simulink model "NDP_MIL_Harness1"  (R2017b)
settings: Solver=FixedStepDiscrete  StartTime=0.0  StopTime=70  FixedStep=0.01  RelTol=1e-3  EnableMultiTasking=on
undefined symbols (not defined in the file): sigbuilder_block

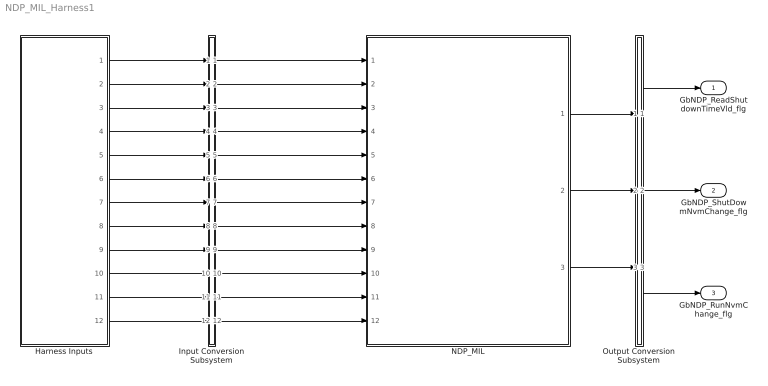
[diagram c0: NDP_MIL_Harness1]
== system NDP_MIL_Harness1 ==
  Harness Inputs : Subsystem  Tag=STV Subsys  LoadFcn=sigbuilder_block('load');  StartFcn=sigbuilder_block('start');  StopFcn=sigbuilder_block('stop');  ClipboardFcn=sigbuilder_block('clipboard');  mask(Sigbuilder block){tuvar=[0:10]}
      mask init:
      | if ~strcmp(get_param(bdroot(gcb),'SimulationStatus'),'stopped'),tuvar = sigbuilder_block('maskInit'); end
  Input Conversion Subsystem : Subsystem  Tag=__SLT_ICS__  Description=Signal spec. and routing
  NDP_MIL : ModelReference  ModelNameDialog=NDP_MIL  SimulationMode=Normal  ModelReferenceVersion='M115C124'
  Output Conversion Subsystem : Subsystem  Tag=__SLT_OCS__  Description=Signal spec. and routing
  GbNDP_ReadShutdownTimeVld_flg : Outport  OutDataTypeStr=boolean  PortDimensions=[1]
  GbNDP_ShutDowmNvmChange_flg : Outport  Port=2  OutDataTypeStr=boolean  PortDimensions=[1]
  GbNDP_RunNvmChange_flg : Outport  Port=3  OutDataTypeStr=boolean  PortDimensions=[1]
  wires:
  Harness Inputs/1(GbNVM_ReadTimeYrVld_flg) -> Input Conversion Subsystem/1(Inport_1)
  Harness Inputs/2(GbNVM_ReadTimeMonthVld_flg) -> Input Conversion Subsystem/2(Inport_2)
  Harness Inputs/3(GbNVM_ReadTimeDayVld_flg) -> Input Conversion Subsystem/3(Inport_3)
  Harness Inputs/4(GbNVM_ReadTimeHrVld_flg) -> Input Conversion Subsystem/4(Inport_4)
  Harness Inputs/5(GbNVM_ReadTimeMintVld_flg) -> Input Conversion Subsystem/5(Inport_5)
  Harness Inputs/6(GbNVM_ReadTimeSecVld_flg) -> Input Conversion Subsystem/6(Inport_6)
  Harness Inputs/7(GeMSM_BMUState_enum) -> Input Conversion Subsystem/7(Inport_7)
  Harness Inputs/8(GbACC_ACChrgFinish_flg) -> Input Conversion Subsystem/8(Inport_8)
  Harness Inputs/9(GbDCC_DCChrgFinish_flg) -> Input Conversion Subsystem/9(Inport_9)
  Harness Inputs/10(GeCTC_CtrCtlState_enum) -> Input Conversion Subsystem/10(Inport_10)
  Harness Inputs/11(GbDAS_HVSafetyNVMStore_flg) -> Input Conversion Subsystem/11(Inport_11)
  Harness Inputs/12(GbDAS_NormalNVMStore_flg) -> Input Conversion Subsystem/12(Inport_12)
  Output Conversion Subsystem/1(Outport_1) -> GbNDP_ReadShutdownTimeVld_flg/1
  Output Conversion Subsystem/2(Outport_2) -> GbNDP_ShutDowmNvmChange_flg/1
  Output Conversion Subsystem/3(Outport_3) -> GbNDP_RunNvmChange_flg/1
  Input Conversion Subsystem/1(Outport_1) -> NDP_MIL/1
  Input Conversion Subsystem/2(Outport_2) -> NDP_MIL/2
  Input Conversion Subsystem/3(Outport_3) -> NDP_MIL/3
  Input Conversion Subsystem/4(Outport_4) -> NDP_MIL/4
  Input Conversion Subsystem/5(Outport_5) -> NDP_MIL/5
  Input Conversion Subsystem/6(Outport_6) -> NDP_MIL/6
  Input Conversion Subsystem/7(Outport_7) -> NDP_MIL/7
  Input Conversion Subsystem/8(Outport_8) -> NDP_MIL/8
  Input Conversion Subsystem/9(Outport_9) -> NDP_MIL/9
  Input Conversion Subsystem/10(Outport_10) -> NDP_MIL/10
  Input Conversion Subsystem/11(Outport_11) -> NDP_MIL/11
  Input Conversion Subsystem/12(Outport_12) -> NDP_MIL/12
  NDP_MIL/1 -> Output Conversion Subsystem/1(Inport_1)
  NDP_MIL/2 -> Output Conversion Subsystem/2(Inport_2)
  NDP_MIL/3 -> Output Conversion Subsystem/3(Inport_3)

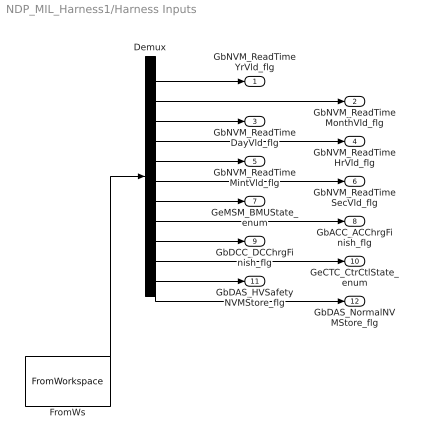
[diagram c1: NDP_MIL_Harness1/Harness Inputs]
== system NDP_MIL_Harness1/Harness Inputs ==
  Demux : Demux  Tag=STV Demux  Outputs=12
  FromWs : FromWorkspace  Tag=STV FromWs  VariableName=tuvar  SampleTime=0
  GbNVM_ReadTimeYrVld_flg : Outport  Tag=STV Outport
  GbNVM_ReadTimeMonthVld_flg : Outport  Tag=STV Outport  Port=2
  GbNVM_ReadTimeDayVld_flg : Outport  Tag=STV Outport  Port=3
  GbNVM_ReadTimeHrVld_flg : Outport  Tag=STV Outport  Port=4
  GbNVM_ReadTimeMintVld_flg : Outport  Tag=STV Outport  Port=5
  GbNVM_ReadTimeSecVld_flg : Outport  Tag=STV Outport  Port=6
  GeMSM_BMUState_enum : Outport  Tag=STV Outport  Port=7
  GbACC_ACChrgFinish_flg : Outport  Tag=STV Outport  Port=8
  GbDCC_DCChrgFinish_flg : Outport  Tag=STV Outport  Port=9
  GeCTC_CtrCtlState_enum : Outport  Tag=STV Outport  Port=10
  GbDAS_HVSafetyNVMStore_flg : Outport  Tag=STV Outport  Port=11
  GbDAS_NormalNVMStore_flg : Outport  Tag=STV Outport  Port=12
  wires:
  FromWs/1 -> Demux/1
  Demux/1 -> GbNVM_ReadTimeYrVld_flg/1
  Demux/2 -> GbNVM_ReadTimeMonthVld_flg/1
  Demux/3 -> GbNVM_ReadTimeDayVld_flg/1
  Demux/4 -> GbNVM_ReadTimeHrVld_flg/1
  Demux/5 -> GbNVM_ReadTimeMintVld_flg/1
  Demux/6 -> GbNVM_ReadTimeSecVld_flg/1
  Demux/7 -> GeMSM_BMUState_enum/1
  Demux/8 -> GbACC_ACChrgFinish_flg/1
  Demux/9 -> GbDCC_DCChrgFinish_flg/1
  Demux/10 -> GeCTC_CtrCtlState_enum/1
  Demux/11 -> GbDAS_HVSafetyNVMStore_flg/1
  Demux/12 -> GbDAS_NormalNVMStore_flg/1

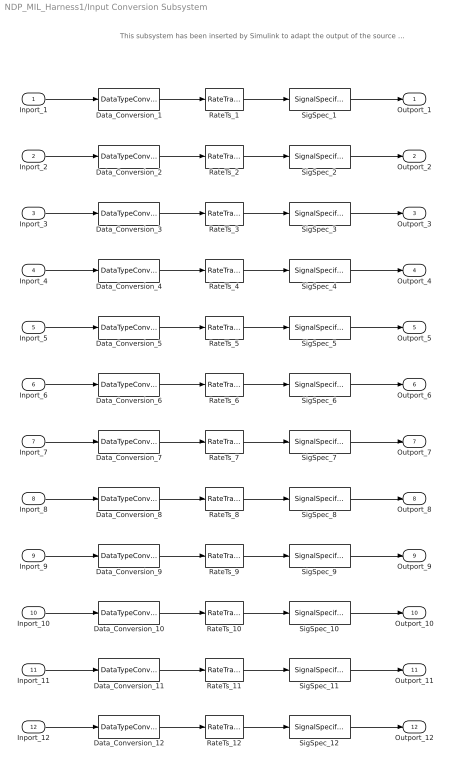
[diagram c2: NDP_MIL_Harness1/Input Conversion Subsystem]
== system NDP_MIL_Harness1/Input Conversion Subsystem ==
  note: This subsystem has been inserted by Simulink to adapt the output of the source blocks to the interface required by the harnessed component. Modifying the contents of this subsystem may result in compilation and simulation failure.
  Inport_1 : Inport
  Inport_2 : Inport  Port=2
  Inport_3 : Inport  Port=3
  Inport_4 : Inport  Port=4
  Inport_5 : Inport  Port=5
  Inport_6 : Inport  Port=6
  Inport_7 : Inport  Port=7
  Inport_8 : Inport  Port=8
  Inport_9 : Inport  Port=9
  Inport_10 : Inport  Port=10
  Inport_11 : Inport  Port=11
  Inport_12 : Inport  Port=12
  Data_Conversion_{1..6,8..9,11..12} (10 alike) : DataTypeConversion  OutDataTypeStr=boolean
  Data_Conversion_10 : DataTypeConversion  OutDataTypeStr=uint8
  Data_Conversion_7 : DataTypeConversion  OutDataTypeStr=uint8
  RateTs_{1..12} (12 alike) : RateTransition  OutPortSampleTime=0.01
  SigSpec_{1..6,8..9} (8 alike) : SignalSpecification  OutDataTypeStr=boolean  Unit=flag  Dimensions=[1]  SampleTime=0.01
  SigSpec_10 : SignalSpecification  OutDataTypeStr=uint8  Unit=enum  Dimensions=[1]  SampleTime=0.01
  SigSpec_11 : SignalSpecification  OutDataTypeStr=boolean  Unit=numb  Dimensions=[1]  SampleTime=0.01
  SigSpec_12 : SignalSpecification  OutDataTypeStr=boolean  Unit=numb  Dimensions=[1]  SampleTime=0.01
  SigSpec_7 : SignalSpecification  OutDataTypeStr=uint8  Unit=enum  Dimensions=[1]  SampleTime=0.01
  Outport_1 : Outport
  Outport_2 : Outport  Port=2
  Outport_3 : Outport  Port=3
  Outport_4 : Outport  Port=4
  Outport_5 : Outport  Port=5
  Outport_6 : Outport  Port=6
  Outport_7 : Outport  Port=7
  Outport_8 : Outport  Port=8
  Outport_9 : Outport  Port=9
  Outport_10 : Outport  Port=10
  Outport_11 : Outport  Port=11
  Outport_12 : Outport  Port=12
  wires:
  SigSpec_1/1 -> Outport_1/1
  RateTs_1/1 -> SigSpec_1/1
  Data_Conversion_1/1 -> RateTs_1/1
  Inport_1/1 -> Data_Conversion_1/1
  SigSpec_2/1 -> Outport_2/1
  RateTs_2/1 -> SigSpec_2/1
  Data_Conversion_2/1 -> RateTs_2/1
  Inport_2/1 -> Data_Conversion_2/1
  SigSpec_3/1 -> Outport_3/1
  RateTs_3/1 -> SigSpec_3/1
  Data_Conversion_3/1 -> RateTs_3/1
  Inport_3/1 -> Data_Conversion_3/1
  SigSpec_4/1 -> Outport_4/1
  RateTs_4/1 -> SigSpec_4/1
  Data_Conversion_4/1 -> RateTs_4/1
  Inport_4/1 -> Data_Conversion_4/1
  SigSpec_5/1 -> Outport_5/1
  RateTs_5/1 -> SigSpec_5/1
  Data_Conversion_5/1 -> RateTs_5/1
  Inport_5/1 -> Data_Conversion_5/1
  SigSpec_6/1 -> Outport_6/1
  RateTs_6/1 -> SigSpec_6/1
  Data_Conversion_6/1 -> RateTs_6/1
  Inport_6/1 -> Data_Conversion_6/1
  SigSpec_7/1 -> Outport_7/1
  RateTs_7/1 -> SigSpec_7/1
  Data_Conversion_7/1 -> RateTs_7/1
  Inport_7/1 -> Data_Conversion_7/1
  SigSpec_8/1 -> Outport_8/1
  RateTs_8/1 -> SigSpec_8/1
  Data_Conversion_8/1 -> RateTs_8/1
  Inport_8/1 -> Data_Conversion_8/1
  SigSpec_9/1 -> Outport_9/1
  RateTs_9/1 -> SigSpec_9/1
  Data_Conversion_9/1 -> RateTs_9/1
  Inport_9/1 -> Data_Conversion_9/1
  SigSpec_10/1 -> Outport_10/1
  RateTs_10/1 -> SigSpec_10/1
  Data_Conversion_10/1 -> RateTs_10/1
  Inport_10/1 -> Data_Conversion_10/1
  SigSpec_11/1 -> Outport_11/1
  RateTs_11/1 -> SigSpec_11/1
  Data_Conversion_11/1 -> RateTs_11/1
  Inport_11/1 -> Data_Conversion_11/1
  SigSpec_12/1 -> Outport_12/1
  RateTs_12/1 -> SigSpec_12/1
  Data_Conversion_12/1 -> RateTs_12/1
  Inport_12/1 -> Data_Conversion_12/1

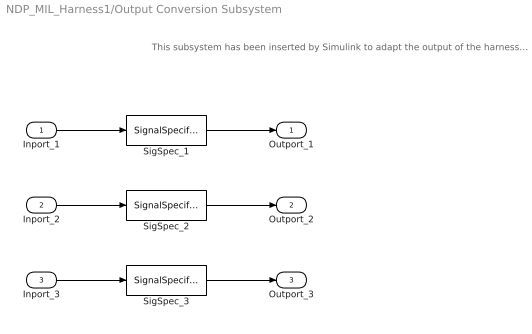
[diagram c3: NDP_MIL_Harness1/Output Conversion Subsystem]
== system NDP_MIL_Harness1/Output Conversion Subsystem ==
  note: This subsystem has been inserted by Simulink to adapt the output of the harnessed component to the interface required by the sink blocks. Modifying the contents of this subsystem may result in compilation and simulation failure.
  Inport_1 : Inport
  Inport_2 : Inport  Port=2
  Inport_3 : Inport  Port=3
  SigSpec_1 : SignalSpecification  OutDataTypeStr=boolean  Unit=flag  Dimensions=[1]  SampleTime=0.01
  SigSpec_2 : SignalSpecification  OutDataTypeStr=boolean  Unit=flag  Dimensions=[1]  SampleTime=0.01
  SigSpec_3 : SignalSpecification  OutDataTypeStr=boolean  Unit=flag  Dimensions=[1]  SampleTime=0.01
  Outport_1 : Outport
  Outport_2 : Outport  Port=2
  Outport_3 : Outport  Port=3
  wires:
  Inport_1/1 -> SigSpec_1/1
  SigSpec_1/1 -> Outport_1/1
  Inport_2/1 -> SigSpec_2/1
  SigSpec_2/1 -> Outport_2/1
  Inport_3/1 -> SigSpec_3/1
  SigSpec_3/1 -> Outport_3/1
